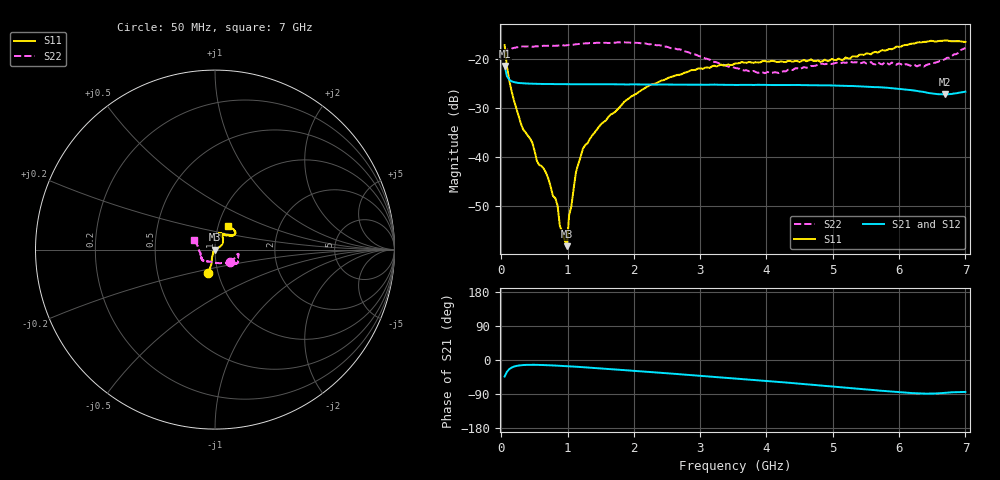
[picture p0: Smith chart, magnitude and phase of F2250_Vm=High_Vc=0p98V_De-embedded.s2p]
! Integrated Device Technology
! Corporate Headquarters
! 6024 Silver Creek Valley Road
! San Jose, CA 95138  USA
! Phone:  1-408-284-8200
! Toll Free:  1-800-223-1366
! Webpage:  http://www.idt.com/
! Timing and RF Division
! 515 Groton Road, Suite 102
! Westford, MA 01886-6024
! Device:  F2250
! Description: Voltage Variable RF Attenuator
! Frequency:  50.0 -  6000.00 MHz
! Package:  3x3 mm Thin QFN Plastic Package: 16 pin
! Ports:  2 RF, 3 DC
!  Pin  1  = GND
!  Pin  2  = NC
!  Pin  3  = RF1  = Port 1
!  Pin  4  = NC
!  Pin  5  = GND
!  Pin  6  = GND
!  Pin  7  = GND
!  Pin  8  = GND
!  Pin  9  = NC
!  Pin 10  = RF2  = Port 2
!  Pin 11  = NC
!  Pin 12  = GND
!  Pin 13  = GND
!  Pin 14  = VCNTRL
!  Pin 15  = VDD
!  Pin 16  = VMODE
! Vcntrl:  0.980 Volts
! Vmode:  +3.300 Volts
! Vdd:  +3.30  Volts
! Current:  1.321 mA
! Data:  The device was measured on a the F2250 evaluation board which has
!  individual transmission lines to the RF pins.  Data was collected
!  using a calibrated network analyzer.  The evaluation board was
!  de-embedded using a TRL calibration technique.
!  The reference plane is the edge of the package pin.
! Misc:  SN 10
!  Action Tracker AT0258
! Date Measured:  2014-11-26
! Date:  2015-10-15  MJV
! Note:
!  Integrated Device Technology supplies this data as a sample of measured
!  data at the package pin for this product.  Your particular data for this
!  product may vary.
!  Data was taken at 25 degrees C.
!  Integrated Device Technology reserves the right to change this data at anytime.
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# GHz S dB R 50
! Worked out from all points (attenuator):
!   201 points, 50 MHz to 7 GHz, reference 50 ohm
!   highest |S21| = -21.47 dB at 50 MHz (marker M1); lowest = -27.3 dB at 6.687 GHz (marker M2)
!   lowest |S11| = -58.2 dB at 988.2 MHz (marker M3), VSWR 1.00, Z = 50.1 - j0.0695 ohm
!   |S11| at or under -10 dB: start of sweep to end of sweep
!   |S22| runs from -23.0 to -16.7 dB; largest |S21 - S12| = 0.00025
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0.05  -17.24 -106.0  -21.47 -43.7  -21.47 -43.7  -19.29 -41.1
0.1195  -24.41 -107.2  -24.29 -24.2  -24.29 -24.2  -18.04 -14.3
0.29325  -33.12 -115.8  -24.99 -13.9  -25.00 -13.9  -17.53 -10.9
0.467  -37.09 -131.3  -25.10 -12.7  -25.11 -12.7  -17.57 -11.4
0.5365  -40.82 -135.3  -25.14 -12.8  -25.13 -12.8  -17.48 -12.7
0.71025  -44.47 -145.1  -25.16 -13.8  -25.17 -13.8  -17.38 -15.7
0.84925  -49.94 -179.5  -25.18 -15.0  -25.17 -15.0  -17.35 -18.5
0.884  -54.15 172.5  -25.19 -15.3  -25.20 -15.3  -17.31 -19.4
0.98825  -58.22 -34.4  -25.21 -16.3  -25.20 -16.3  -17.28 -20.7
1.023  -51.91 1.8  -25.20 -16.6  -25.22 -16.6  -17.20 -20.9
1.05775  -50.01 13.2  -25.23 -17.0  -25.22 -17.0  -17.18 -21.1
1.12725  -43.06 16.2  -25.21 -17.7  -25.19 -17.7  -17.07 -22.6
1.2315  -38.33 18.4  -25.19 -18.9  -25.19 -18.9  -16.92 -24.5
1.857  -28.75 31.8  -25.25 -26.8  -25.26 -26.8  -16.69 -30.7
2.37825  -24.72 41.7  -25.27 -33.4  -25.28 -33.5  -17.23 -35.5
3.525  -20.98 69.5  -25.36 -48.8  -25.36 -48.8  -21.89 -70.8
4.18525  -20.67 75.9  -25.37 -57.8  -25.38 -57.9  -22.93 -110.8
4.7065  -20.46 70.8  -25.41 -65.6  -25.43 -65.6  -21.50 -130.5
5.85325  -18.03 39.4  -25.98 -82.9  -25.99 -83.0  -21.20 -148.8
6.3745  -16.59 40.1  -26.80 -88.7  -26.82 -88.7  -21.62 -168.5
6.68725  -16.31 47.0  -27.31 -86.7  -27.34 -86.8  -20.15 168.2
7  -16.60 61.9  -26.74 -84.3  -26.74 -84.4  -17.82 156.6
